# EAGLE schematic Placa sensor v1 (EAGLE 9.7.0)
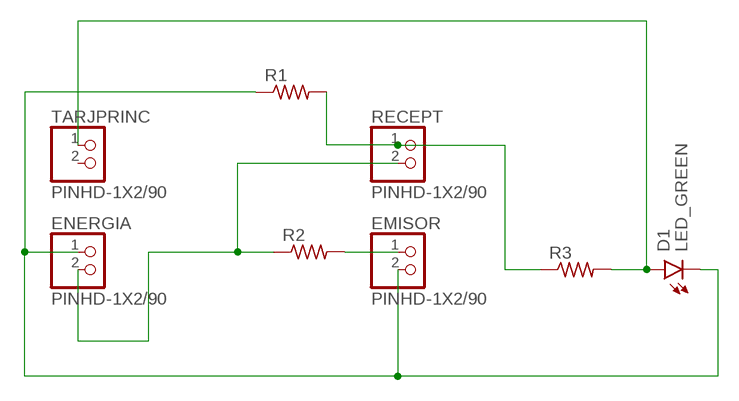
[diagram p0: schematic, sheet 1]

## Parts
D1  LED_GREEN  CHIP-ROUND-G_1209  [LEDC3224X250N_RND-G]
EMISOR  PINHD-1X2/90  [1X02/90]
ENERGIA  PINHD-1X2/90  [1X02/90]
R1  RES-US1206FAB  [R1206FAB]
R2  RES-US1206FAB  [R1206FAB]
R3  RES-US1206FAB  [R1206FAB]
RECEPT  PINHD-1X2/90  [1X02/90]
TARJPRINC  PINHD-1X2/90  [1X02/90]

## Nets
N$1: ENERGIA.2 R2.1 RECEPT.2
N$2: EMISOR.1 R2.2
N$3: D1.C EMISOR.2 ENERGIA.1 R1.1
N$4: R1.2 R3.1 RECEPT.1
N$5: D1.A R3.2 TARJPRINC.1
Unconnected: TARJPRINC.2

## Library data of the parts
D1 = LED:CHIP-ROUND-G; CATEGORY: LED; COLOR: GREEN; DESCRIPTION: CHIP LED ROUND; SUB-CATEGORY: CHIP; TYPE: ROUND_TOP
EMISOR ENERGIA RECEPT TARJPRINC = Connector:PINHD-1X2: PIN HEADER; CATEGORY: CONNECTOR; SUB-CATEGORY: PIN-HEADER
R1-R3 = fab:RES-US: Resistor (US Symbol)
